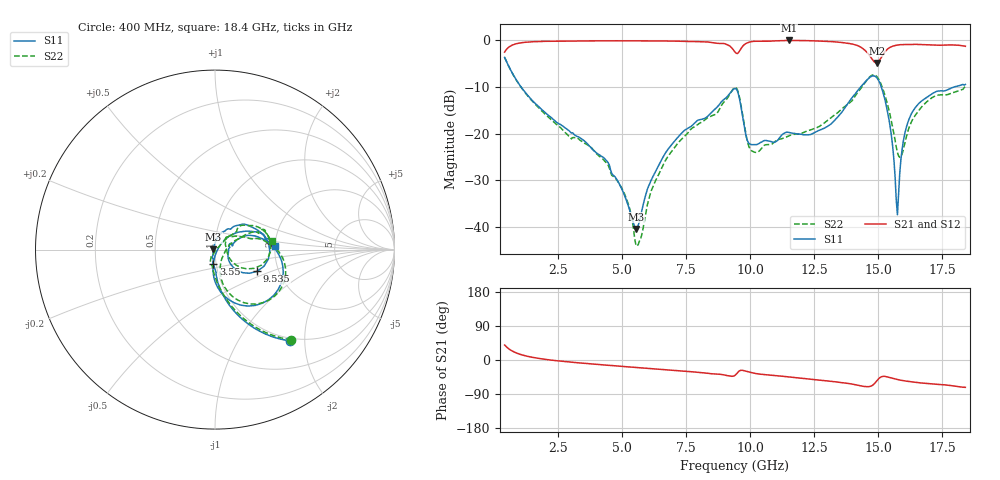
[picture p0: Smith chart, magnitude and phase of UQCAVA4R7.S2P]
!  Part Number  UQCAVA4R7
!  Description: RF capacitor  Mounting Orientation: Horizontal
!  Application:
# GHZ S DB R 50
! Freq  |S11|  S11 Ph  |S21|  S21 Ph  |S12|  S12 Ph  |S22|  S22 Ph
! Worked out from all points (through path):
!   401 points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, 400 MHz to 18.4 GHz, reference 50 ohm
!   highest |S21| = 0.00 dB at 11.52 GHz (marker M1); lowest = -4.8 dB at 14.94 GHz (marker M2)
!   group delay of S21, straight-line fit = 12.6 ps
!   lowest |S11| = -40.5 dB at 5.53 GHz (marker M3), VSWR 1.02, Z = 49.1 + j0.208 ohm
!   |S11| at or under -10 dB: 1.043 GHz to 14.31 GHz (13.27 GHz wide, 173 % of centre); 15.12 GHz to 17.96 GHz (2.841 GHz wide, 17.2 % of centre)
!   |S22| runs from -44.2 to -3.6 dB; largest |S21 - S12| = 0.0024
!   S11 on the Smith chart (normalised r, x): 400 MHz: 0.95, -1.70; 3.55 GHz: 0.97, -0.16; 9.535 GHz: 1.55, -0.40; 18.4 GHz: 2.01, +0.10
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0.4  -3.64 -50.7  -2.50 39.5  -2.49 39.5  -3.64 -49.8
1.165  -10.88 -77.9  -0.41 11.9  -0.41 11.8  -10.96 -77.1
3.415  -21.16 -94.3  -0.10 -8.4  -0.09 -8.4  -21.68 -104.4
3.55  -21.78 -95.9  -0.11 -9.2  -0.10 -9.3  -22.17 -105.9
4.99  -32.09 -116.0  -0.08 -16.9  -0.08 -16.9  -31.86 -110.0
5.53  -40.49 167.1  -0.10 -19.5  -0.10 -19.6  -43.93 -65.1
6.43  -26.70 86.1  -0.11 -24.2  -0.11 -24.3  -28.66 40.7
8.86  -13.24 40.3  -0.64 -38.0  -0.65 -38.0  -14.05 42.8
9.4  -10.30 -2.0  -2.50 -40.5  -2.51 -40.6  -10.09 6.4
9.535  -11.57 -27.3  -2.62 -30.8  -2.63 -30.8  -11.27 -18.5
9.85  -20.88 -34.8  -0.59 -29.9  -0.60 -30.0  -20.83 -29.7
10.075  -22.39 -9.2  -0.22 -33.7  -0.23 -33.8  -23.79 1.2
11.515  -19.78 14.1  0.00 -44.9  0.00 -45.0  -20.48 47.9
12.415  -20.07 17.2  -0.08 -51.0  -0.08 -51.0  -19.09 40.1
14.125  -11.27 12.7  -0.98 -65.5  -0.99 -65.5  -11.68 12.9
14.665  -7.93 -18.7  -3.29 -69.8  -3.29 -69.8  -7.81 -15.0
14.935  -7.99 -48.5  -4.81 -55.4  -4.82 -55.4  -7.71 -43.2
15.43  -17.49 -94.1  -1.57 -46.1  -1.58 -46.1  -15.30 -78.0
15.745  -37.46 -13.8  -0.98 -51.5  -0.99 -51.5  -24.08 -51.9
16.015  -20.48 44.2  -0.88 -55.0  -0.88 -55.0  -22.49 12.6
16.375  -14.97 33.9  -0.85 -58.1  -0.85 -58.1  -16.63 24.6
18.4  -9.45 3.8  -1.25 -72.3  -1.25 -72.2  -9.92 8.6
